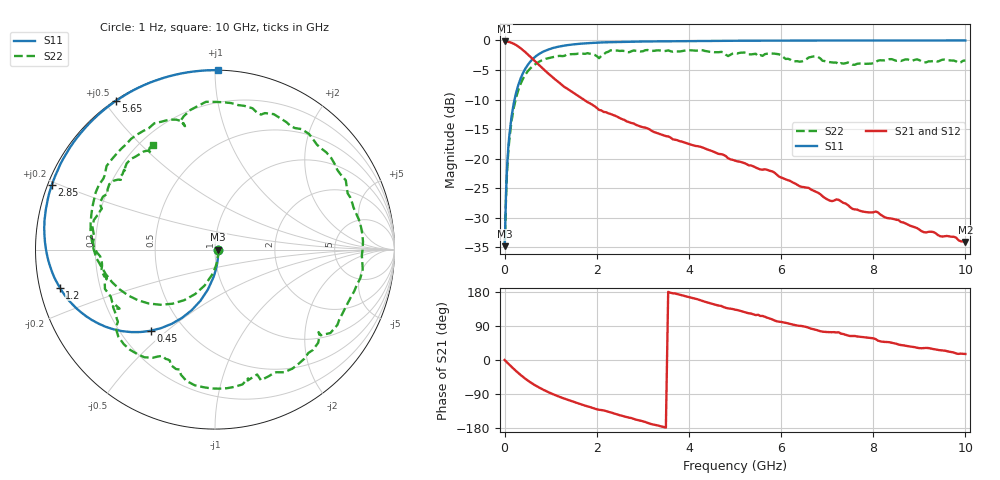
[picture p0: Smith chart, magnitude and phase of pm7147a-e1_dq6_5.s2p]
# GHz S DB R 50
! S-Parameters data
! Freq  dbS11  angS11  dbS21  angS21  dbS12  angS12  dbS22  angS22
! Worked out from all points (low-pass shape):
!   279 points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, 1 Hz to 10 GHz, reference 50 ohm
!   highest |S21| = -0.16 dB at 125.9 Hz (marker M1); lowest = -34.0 dB at 10 GHz (marker M2)
!   |S21| within 3 dB of the highest: start of sweep to 611.9 MHz
!   lowest |S11| = -34.8 dB at 125.9 Hz (marker M3), VSWR 1.04, Z = 51.9 - j1e-05 ohm
!   |S11| at or under -10 dB: start of sweep to 216.2 MHz
!   |S22| runs from -34.8 to -1.6 dB; largest |S21 - S12| = 0
!   S11 on the Smith chart (normalised r, x): 1 Hz: 1.04, -0.00; 450 MHz: 0.32, -0.44; 1.2 GHz: 0.06, -0.12; 2.85 GHz: 0.01, +0.19; 5.65 GHz: 0.00, +0.54; 10 GHz: 0.00, +1.02
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1e-09  -34.78 -0.0  -0.16 -0.0  -0.16 -0.0  -34.78 -0.0
1.259e-07  -34.78 -0.0  -0.16 -0.0  -0.16 -0.0  -34.78 -0.0
0.03162278  -25.67 -72.3  -0.17 -3.8  -0.17 -3.8  -26.31 -72.0
0.06309573  -20.12 -85.4  -0.21 -7.6  -0.21 -7.6  -20.83 -87.1
0.15  -12.89 -100.1  -0.39 -17.9  -0.39 -17.9  -13.64 -106.1
0.3  -7.47 -115.8  -1.04 -34.6  -1.04 -34.6  -8.32 -128.2
0.45  -4.77 -128.4  -1.98 -49.4  -1.98 -49.4  -5.78 -146.7
0.8  -2.05 -150.2  -4.54 -76.0  -4.54 -76.0  -3.39 179.8
1.2  -1.01 -166.2  -7.22 -97.7  -7.22 -97.7  -2.61 150.9
1.7  -0.52 180.0  -9.91 -118.5  -9.91 -118.5  -2.24 121.1
2.3  -0.29 167.7  -12.44 -138.2  -12.44 -138.2  -1.67 93.5
2.85  -0.19 158.4  -14.26 -157.4  -14.26 -157.4  -1.75 63.5
3.35  -0.14 151.0  -15.75 -173.7  -15.75 -173.7  -1.68 38.1
4.25  -0.08 139.2  -17.98 157.7  -17.98 157.7  -1.62 -7.6
5.05  -0.05 130.0  -20.44 131.8  -20.44 131.8  -2.20 -47.9
5.65  -0.04 123.6  -21.78 114.1  -21.78 114.1  -2.31 -78.5
6.05  -0.03 119.7  -23.31 99.3  -23.31 99.3  -2.83 -105.3
6.7  -0.02 113.6  -25.39 81.3  -25.39 81.3  -2.71 -130.3
6.9  -0.02 111.8  -26.34 74.7  -26.34 74.7  -3.43 -143.4
8.35  -0.01 100.2  -30.07 46.9  -30.07 46.9  -3.17 169.5
9  -0.00 95.6  -31.99 31.3  -31.99 31.3  -3.33 145.6
10  -0.00 89.1  -34.05 15.9  -34.05 15.9  -3.38 120.7
